FUNCTION_BLOCK FB14
TITLE =Get Position Regulation Gain
//*****************************************************************************
//* maxon motor ag
//* R&D
//* all rights reserved
//*****************************************************************************
//* Summary:  Read position regulation gains (PID)
//*
//* Remarks:
//*
//* Created under: STEP7 REV5.2+SP1
//*****************************************************************************
//* History:
//* 19.05.2004 | INA   first release
//*
//*
//*****************************************************************************
//

AUTHOR:INA
FAMILY:Configur
NAME:GPosRegG
VERSION:00.01


VAR_INPUT

Read : BOOL //A rising edge start the command

  NodeID : BYTE //Adress of the maxon device

END_VAR
VAR_OUTPUT
  Done : BOOL //Data valid flag is TRUE if data were available

  Err : BOOL //Error flag is TRUE if an Error has occured, see ErrNo for more details

  ErrNo : DINT //Contains detailed error information

  P_Gain : WORD //Position Regulator P-Gain

  I_Gain : WORD //Position Regulator I-Gain

  D_Gain : WORD //Position Regulator D-Gain

END_VAR
VAR
  xEdgeMerker : BOOL //Edge Merker

  xEdgeFlag : BOOL //Edge Flag

  xStep : INT
END_VAR

BEGIN

NETWORK
TITLE = Activate the service function
//

// SDO Read "Get Position Regulation Gain"

       U    #Read
       FP   #xEdgeFlag                   // recognize a positiv edge of the Read signal
       =    #xEdgeMerker                 // and set the xEdgeMerker for one cycle to true

       L    #xStep
       L    0
       ==I
       U    #xEdgeMerker
       SPB  nstp                         // iStep = 1 -> fnc1

       L    #xStep                       // jump list
       SPL  List
       SPA  rdef
       SPA  fnc1
       SPA  fncE
List  :SPA  rdef

rdef  :NOP  0
       R    #Done                        // reset Done
       R    #Err                         // reset Error
       L    0
       T    #xStep                       // iStep = 0
       SPA  end

fnc1  :NOP  0
       CALL FC1
         NodeID:=#NodeID
         Index:=DW#16#000060FB
         SubIndex:=DW#16#00000001
         RET_VAL:=#Done
         Err:=#Err
         ErrNo:=#ErrNo

       L    DB219.DBW10
       T    #P_Gain

       L    1
       U    #Err
       SPB  fncE

       NOP  0
       CALL FC1
         NodeID:=#NodeID
         Index:=DW#16#000060FB
         SubIndex:=DW#16#00000002
         RET_VAL:=#Done
         Err:=#Err
         ErrNo:=#ErrNo

       L    DB219.DBW10
       T    #I_Gain

       L    1
       U    #Err
       SPB  fncE

       NOP  0
       CALL FC1
         NodeID:=#NodeID
         Index:=DW#16#000060FB
         SubIndex:=DW#16#00000003
         RET_VAL:=#Done
         Err:=#Err
         ErrNo:=#ErrNo

       L    DB219.DBW10
       T    #D_Gain

fncE  :NOP  0
       L    0
       T    #xStep
       SPA  end

nstp  :NOP  0
       L    #xStep
       INC            1
       T    #xStep

end   :NOP  0
END_FUNCTION_BLOCK
